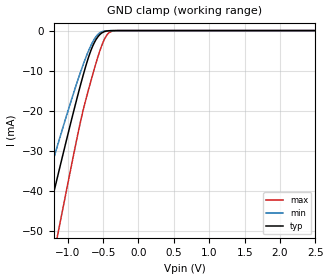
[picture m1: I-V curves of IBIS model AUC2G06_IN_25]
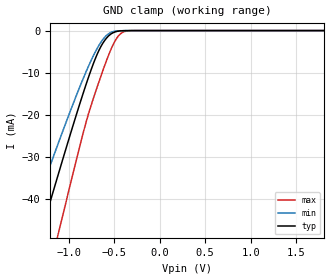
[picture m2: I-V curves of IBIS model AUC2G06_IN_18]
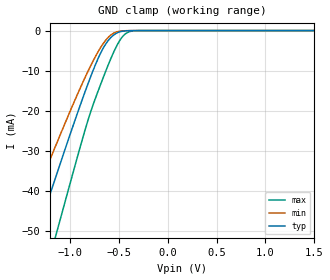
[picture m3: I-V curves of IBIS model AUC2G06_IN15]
| TEXAS INSTRUMENTS INCORPORATED
| Standard Linear and Logic Group
| IBIS Model of SN74AUC2G06
| Dual Inverter Buffer/Driver with Open-Drain Outputs
| This file contains package information for the following:
|  SOT 6-pin (DBV) package as [Component] AUC2G06_DBV
|  SOT 6-pin (DCK) package as [Component] AUC2G06_DCK
| This device can be powered at the following Vccs:
|  2.5 volt Vcc
|  1.8 volt Vcc
|  1.5 volt Vcc
|  1.2 volt Vcc
|  0.8 volt Vcc
| This file provides unique models under the [Model Selector] for each Vcc.
| For operation at a specific Vcc, select the appropriate model after each
| [Model Selector] keyword.
[IBIS Ver]   3.2
[Comment char]  |_char
[File Name]   sn74auc2g06.ibs
[File Rev]   1.1 | x_die
[Date]   November 26, 2002
[Source]   Data created from TI-SPICE simulations at TI-SLL.
[Notes]   The following is an IBIS list for the AUC2G06.
   Please contact sllibis@ti.com with questions and
   comments concerning SLL IBIS models.
   - Non-monotonic data in pulldown due to feedback circuit.
   - End point warning due to AC and DC mismatch.
   - The slow Rising Waveforms in the AUC2G06_OUT are normal for
   this open-drain (TPLZ) device.
[Disclaimer] Property of Texas Instruments Incorporated.  Unauthorized
   reproduction and/or distribution is strictly prohibited.
   This product is protected under copyright law.
   Created  2002, (C) Copyright  2002, Texas Instruments
   Incorporated, All Rights Reserved
   UNLESS THERE IS A SIGNED, WRITTEN AGREEMENT TO THE
   CONTRARY, TEXAS INSTRUMENTS (TI) IS PROVIDING THE IBIS
   MODELS  AND WITHOUT ANY WARRANTY, EXPRESSED OR
   IMPLIED.  TI assumes no liability for:
   1) the accuracy of the IBIS models provided to your
   company;
   2) the proper functioning of these IBIS Models in your
   design or for any resulting applications; or
   3) infringement of patents, copyrights or intellectual
   property rights resulting from your use of these IBIS
   models.
   TI provides IBIS Models as a service to our customers.
   You and your company shall not distribute, sell or give
   these models to anyone else without prior written
   permission from TI.
   TI reserves the right to make changes to our products or
   to discontinue any semiconductor product or service
   without notice, and advises our customers to obtain the
   latest version of relevant information to verify, before
   placing orders, that the information being relied on is
   current.
   Please be aware that your receipt and use of the IBIS
   information provided shall serve as acceptance of these
   terms and conditions.  If you do not accept these terms,
   you should return or destroy the IBIS models and any
   other accompanying information immediately.
| Component AUC2G06_DBV 6-pin SOT
[Component]   AUC2G06_DBV
[Manufacturer]   Texas Instruments, Inc.
[Package]
|   typ   min   max
R_pkg   0.025   0.019   0.037
L_pkg   1.524nH   1.260nH   1.751nH
C_pkg   0.245pF   0.198pF   0.264pF
[Pin]   signal_name   model_name   R_pin   L_pin   C_pin
1   1A   AUC2G06_IN   0.021   1.405nH   0.246pF
2   GND   GND   0.037   1.751nH   0.263pF
3   2A   AUC2G06_IN   0.026   1.493nH   0.247pF
4   2Y   AUC2G06_OUT   0.019   1.620nH   0.264pF
5   VCC   POWER   0.024   1.260nH   0.198pF
6   1Y   AUC2G06_OUT   0.021   1.617nH   0.250pF
| Component AUC2G06_DCK 6-pin SOT
[Component]   AUC2G06_DCK
[Manufacturer]   Texas Instruments, Inc.
[Package]
|   typ   min   max
R_pkg   1.400e-02   1.100e-02   2.100e-02
L_pkg   9.480e-10   7.840e-10   1.103e-09
C_pkg   1.910e-13   1.670e-13   2.050e-13
[Pin]   signal_name   model_name   R_pin   L_pin   C_pin
1   1A   AUC2G06_IN   1.300e-02   9.840e-10   1.960e-13
2   GND   GND   2.100e-02   1.103e-09   2.050e-13
3   2A   AUC2G06_IN   1.100e-02   9.980e-10   1.970e-13
4   2Y   AUC2G06_OUT   1.300e-02   9.040e-10   1.900e-13
5   VCC   POWER   1.500e-02   7.840e-10   1.670e-13
6   1Y   AUC2G06_OUT   1.200e-02   9.160e-10   1.950e-13
| Model AUC2G06_IN
[Model Selector]   AUC2G06_IN
AUC2G06_IN_25   2.5 volt Vcc
AUC2G06_IN_18   1.8 volt Vcc
AUC2G06_IN15   1.5 volt Vcc
AUC2G06_IN_12   1.2 volt Vcc
AUC2G06_IN_08   0.8 volt Vcc
| Model AUC2G06_OUT
[Model Selector]   AUC2G06_OUT
AUC2G06_OUT_25   2.5 volt Vcc
AUC2G06_OUT_18   1.8 volt Vcc
AUC2G06_OUT15   1.5 volt Vcc
AUC2G06_OUT_12   1.2 volt Vcc
AUC2G06_OUT_08   0.8 volt Vcc
| Models and submodels in the file (10): AUC2G06_IN_25 (Input), AUC2G06_IN_18 (Input), AUC2G06_IN15 (Input), AUC2G06_IN_12 (Input), AUC2G06_IN_08 (Input), AUC2G06_OUT_25 (Open_drain), AUC2G06_OUT_18 (Open_drain), AUC2G06_OUT15 (Open_drain), AUC2G06_OUT_12 (Open_drain), AUC2G06_OUT_08 (Open_drain)
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[Model]   AUC2G06_IN_25
Model_type  Input
Vinl=0.7
Vinh=1.7
| variable   typ   min   max
C_comp   2.28pF   1.83pF   2.65pF
[Temperature Range]   40   100   -40
| Ambient temperature   25   85   -40
[Voltage range]   2.5   2.3   2.7
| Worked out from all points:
|   GND clamp passes 1 mA (typ) near -0.55 V on its own axis
[GND Clamp]
| AUC2G06_IN_25
|   Voltage   I(typ)   I(min)   I(max)
-3.6V     -222.3mA   -186.1mA   -267.5mA
-1.49V    -62.29mA   -49.79mA   -82.1mA
-1.35V    -51.8mA    -41.14mA   -69.63mA
-1.305V   -48.45mA   -38.39mA   -65.61mA
-1.17V    -38.46mA   -30.25mA   -53.55mA
-1.12V    -34.79mA   -27.28mA   -49.08mA
-735mV    -8.324mA   -6.331mA   -16.67mA
-635mV    -3.426mA   -2.471mA   -10.25mA
-525mV    -682.5uA   -360.4uA   -4.021mA
-430mV    -73.19uA   -34.73uA   -776.9uA
-325mV    -3.339uA   -2.006uA   -30.74uA
2.5V      313.9pA    400.9pA    470.4pA
[Model]   AUC2G06_IN_18
Model_type  Input
Vinl=0.5775
Vinh=1.2675
| variable   typ   min   max
C_comp   2.34pF   1.92pF   2.66pF
[Temperature Range]   40   100   -40
| Ambient temperature   25   85   -40
[Voltage range]   1.8   1.65   1.95
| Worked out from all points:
|   GND clamp passes 1 mA (typ) near -0.55 V on its own axis
[GND Clamp]
| AUC2G06_IN_18
|   Voltage   I(typ)   I(min)   I(max)
-3.6V     -222.3mA   -186.1mA   -267.5mA
-1.475V   -61.16mA   -48.85mA   -80.77mA
-1.43V    -57.79mA   -46.07mA   -76.76mA
-1.295V   -47.7mA    -37.79mA   -64.71mA
-1.145V   -36.62mA   -28.76mA   -51.31mA
-1.095V   -32.97mA   -25.81mA   -46.85mA
-830mV    -14.31mA   -10.96mA   -23.64mA
-685mV    -5.607mA   -4.224mA   -13.41mA
-560mV    -1.272mA   -753.7uA   -5.827mA
-485mV    -290.6uA   -140.2uA   -2.305mA
-420mV    -55.81uA   -26.72uA   -608.5uA
1.8V      203.2pA    297.2pA    235.5pA
[Model]   AUC2G06_IN15
Model_type  Input
Vinl=0.49
Vinh=1.04
| variable   typ   min   max
C_comp   2.38pF   1.96pF   2.66pF
[Temperature Range]   40   100   -40
| Ambient temperature   25   85   -40
[Voltage range]   1.5   1.4   1.6
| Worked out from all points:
|   GND clamp passes 1 mA (typ) near -0.55 V on its own axis
[GND Clamp]
| AUC2G06_IN15
|   Voltage   I(typ)   I(min)   I(max)
-3.6V     -222.3mA   -186.1mA   -267.5mA
-1.505V   -63.42mA   -50.72mA   -83.44mA
-1.325V   -49.94mA   -39.61mA   -67.39mA
-1.17V    -38.46mA   -30.25mA   -53.55mA
-1.12V    -34.79mA   -27.28mA   -49.08mA
-840mV    -14.98mA   -11.48mA   -24.46mA
-695mV    -6.114mA   -4.621mA   -14.06mA
-570mV    -1.487mA   -911.6uA   -6.381mA
-495mV    -364.6uA   -178.8uA   -2.692mA
-430mV    -73.19uA   -34.73uA   -776.9uA
-280mV    -781.4nA   -556.3nA   -5.358uA
1.5V      165.9pA    258.5pA    172.1pA
